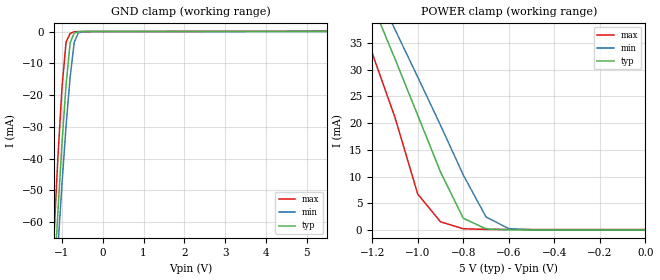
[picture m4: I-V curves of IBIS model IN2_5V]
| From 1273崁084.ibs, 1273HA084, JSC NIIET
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[Model]   IN2_5V
Model_type Input
Polarity   Non-Inverting
Vinl =   0.80V
Vinh =   2.10V
C_comp   1.984800pF   1.899400pF   2.077500pF
[Temperature Range]   25   -60   85
[Voltage Range]   5.00V   4.50V   5.50V
[POWER Clamp Reference]   5.00V   4.50V   5.50V
[GND Clamp Reference]   0.00V   0.00V   0.00V
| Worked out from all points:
|   GND clamp passes 1 mA (typ) near -0.72 V on its own axis
|   POWER clamp passes 1 mA (typ) near -0.74 V on its own axis
[Power Clamp]
| Voltage   I(typ)   I(min)   I(max)
-5.5V     666.5mA    586.4mA    790.2mA
-1.3V     52.63mA    56.46mA    45.01mA
-1.2V     42.3mA     46.72mA    33.09mA
-1.1V     32.03mA    37.52mA    21.08mA
-1V       21.47mA    28.62mA    6.726mA
-900mV    10.86mA    19.6mA     1.537mA
-800mV    2.198mA    10.31mA    227.4uA
-700mV    203.8uA    2.431mA    114.3uA
-600mV    21.74uA    257.9uA    103.7uA
-500mV    8.443uA    25.19uA    101.6uA
0V        7.978uA    4.741uA    97.11uA
[GND Clamp]
| Voltage   I(typ)   I(min)   I(max)
-5.5V     -1.417A    -1.243A    -1.663A
-1.2V     -80.17mA   -89.31mA   -65.26mA
-1.1V     -56.79mA   -68.09mA   -39.71mA
-1V       -35.2mA    -48.04mA   -17.73mA
-900mV    -16.77mA   -29.71mA   -3.319mA
-800mV    -3.55mA    -14.38mA   -611.9uA
-700mV    -481.9uA   -3.406mA   -66.22uA
-600mV    -49.55uA   -442.2uA   -14.05uA
-500mV    -6.288uA   -41.83uA   -9.383uA
5.5V      7.925uA    8.151uA    147.1uA
